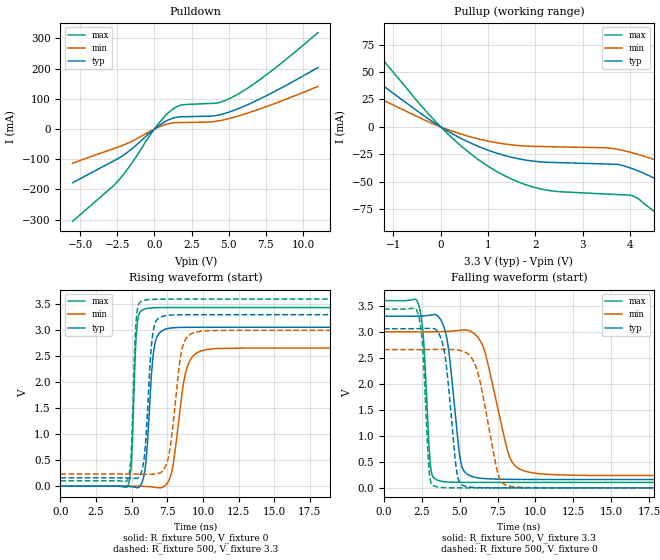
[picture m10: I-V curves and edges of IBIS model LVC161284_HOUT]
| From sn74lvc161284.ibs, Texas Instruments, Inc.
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[Model]   LVC161284_HOUT
Model_type  Output
Vref =   0
Rref =   500
Cref =   50p
Vmeas =   1.5
| variable   typ   min   max
C_comp   3.56pF   1.68pF   5.90pF
| C_pullup   3.41pF   2.14pF   4.10pF
| C_pulldown   3.71pF   1.68pF   5.90pF
[Temperature Range]   40   100   -40
| Ambient temperature   25   85   -40
[Voltage range]   3.3   3   3.6
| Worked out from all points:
|   slope of the pulldown table from 0 to 0.495 V, typ, clamps not added: 27.6 ohm
|   slope of the pullup table from 0 to 0.495 V, typ, clamps not added: 41.7 ohm
|   rising waveform, R_fixture 500, V_fixture 0: 20-80 % time 437ps typ, 766ps min, 266ps max; typ from 0 V to 3.06 V
|   falling waveform, R_fixture 500, V_fixture 3.3: 20-80 % time 667ps typ, 1.28ns min, 373ps max; typ from 3.3 V to 0.161 V
|   rising waveform, R_fixture 500, V_fixture 3.3: 20-80 % time 414ps typ, 677ps min, 258ps max; typ from 0.161 V to 3.3 V
|   falling waveform, R_fixture 500, V_fixture 0: 20-80 % time 604ps typ, 1.05ns min, 356ps max; typ from 3.06 V to 0 V
[Pulldown]
| LVC161284_HOUT
|   Voltage   I(typ)   I(min)   I(max)
-5.5V     -177.6mA   -112.8mA   -305.4mA
-2.435V   -97.24mA   -59.13mA   -170.9mA
-1.59V    -68.03mA   -41.88mA   -117.3mA
145mV     5.682mA    3.501mA    9.654mA
675mV     23.4mA     13.95mA    40.96mA
1.165V    34.8mA     19.84mA    63.26mA
1.885V    40.65mA    21.74mA    80.37mA
4.225V    45.57mA    26.46mA    86.19mA
5.335V    61.71mA    39.02mA    108.1mA
6.375V    83.05mA    54.66mA    139mA
7.64V     113.2mA    76.37mA    183.7mA
11V       203.7mA    141mA      319.5mA
[Pullup]
| LVC161284_HOUT
|   Voltage   I(typ)   I(min)   I(max)
-5.5V     174.8mA    117.5mA    276.7mA
-4.34V    138.3mA    92.57mA    219.8mA
-3.175V   100.9mA    67.07mA    161.1mA
-2.095V   65.8mA     43.4mA     105.8mA
-1.585V   49.29mA    32.33mA    79.56mA
1.12V     -23.01mA   -13.92mA   -38.98mA
2.225V    -32.11mA   -17.95mA   -57.43mA
4.04V     -37.88mA   -23.48mA   -62.54mA
4.9V      -55.04mA   -35.49mA   -90.5mA
6.405V    -91.99mA   -60.48mA   -150.2mA
8.23V     -140.1mA   -92.75mA   -228.5mA
11V       -214.9mA   -142.9mA   -350.8mA
[Ramp]
| LVC161284_HOUT
| variable   typ   min   max
dV/dt_r   1.85/4.49E-10   1.61/7.76E-10   2.08/2.83E-10
dV/dt_f   1.90/6.79E-10   1.68/1.30E-09   2.11/3.83E-10
R_load = 500
[Rising Waveform]
| LVC161284_HOUT
R_fixture =   500
C_fixture =   0
L_fixture =   0
V_fixture =   0
V_fixture_min = 0
V_fixture_max = 0
|   Time   V(typ)   V(min)   V(max)
0s        81.15pV    6.348nV    51.4pV
4.735ns   -3.811mV   664.7uV    12.32mV
4.98ns    -11.31mV   1.045mV    477.8mV
5.38ns    -29.97mV   1.252mV    3.11V
5.99ns    448.7mV    -5.816mV   3.416V
6.585ns   2.674V     -19.33mV   3.434V
7.52ns    3.034V     65.91mV    3.438V
8.83ns    3.057V     2.234V     3.438V
10.11ns   3.058V     2.621V     3.438V
50ns      3.059V     2.658V     3.438V
[Falling Waveform]
| LVC161284_HOUT
R_fixture =   500
C_fixture =   0
L_fixture =   0
V_fixture =   3.3
V_fixture_min = 3
V_fixture_max = 3.6
|   Time   V(typ)   V(min)   V(max)
0s        3.3V       3V         3.6V
2.29ns    3.302V     2.998V     3.515V
2.6ns     3.307V     2.999V     2.895V
3.085ns   3.322V     2.999V     385.8mV
3.715ns   3.247V     3.003V     131.5mV
5.08ns    478.3mV    3.031V     106.1mV
5.985ns   204mV      2.958V     104.8mV
8.295ns   163.6mV    593.7mV    104.4mV
9.575ns   161.5mV    301.3mV    104.4mV
50ns      160.7mV    234.5mV    104.4mV
[Rising Waveform]
| LVC161284_HOUT
R_fixture =   500
C_fixture =   0
L_fixture =   0
V_fixture =   3.3
V_fixture_min = 3
V_fixture_max = 3.6
|   Time   V(typ)   V(min)   V(max)
0s        160.7mV    234.5mV    104.4mV
4.71ns    156.2mV    234.8mV    125mV
4.955ns   152.1mV    234.5mV    583.1mV
5.33ns    151.7mV    233.3mV    3.237V
5.885ns   568.1mV    227.8mV    3.577V
6.48ns    2.936V     230.4mV    3.595V
7.28ns    3.276V     335.4mV    3.599V
8.53ns    3.299V     2.637V     3.6V
9.53ns    3.3V       2.968V     3.6V
50ns      3.3V       3V         3.6V
[Falling Waveform]
| LVC161284_HOUT
R_fixture =   500
C_fixture =   0
L_fixture =   0
V_fixture =   0
V_fixture_min = 0
V_fixture_max = 0
|   Time   V(typ)   V(min)   V(max)
0s        3.059V     2.658V     3.438V
2.25ns    3.062V     2.657V     3.345V
2.545ns   3.064V     2.658V     2.731V
2.995ns   3.065V     2.66V      280.5mV
3.485ns   3.026V     2.663V     20.66mV
4.055ns   2.491V     2.663V     3.793mV
4.83ns    265.1mV    2.651V     652.6uV
5.435ns   26.17mV    2.596V     211.3uV
8.315ns   372.7uV    30.31mV    2.482uV
50ns      81.06pV    6.348nV    50.9pV
